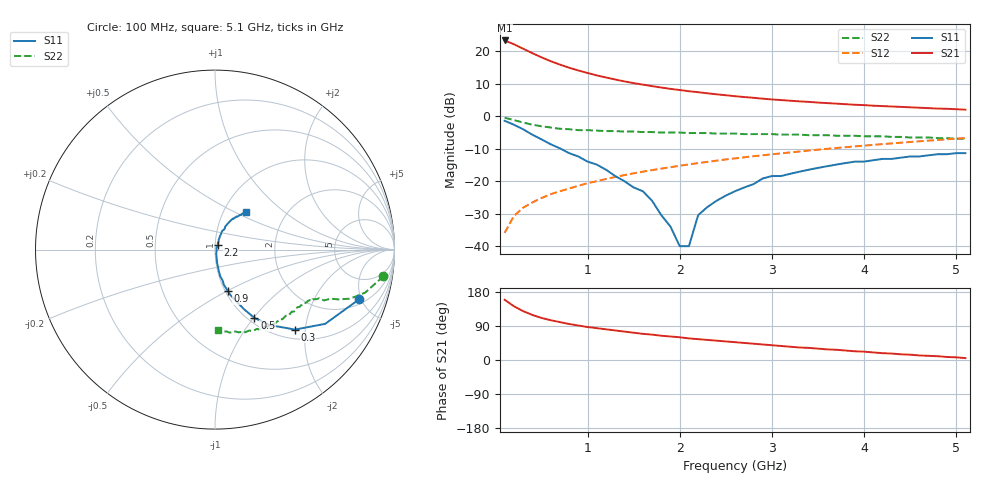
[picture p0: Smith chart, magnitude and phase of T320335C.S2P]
!AT-32033
!S PARAMETERS at Vce=5 V  Ic=5mA.  LAST UPDATED 01-05-95
# ghz s ma r 50
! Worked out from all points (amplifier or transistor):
!   51 points, 100 MHz to 5.1 GHz, reference 50 ohm
!   highest |S21| = 23.3 dB at 100 MHz (marker M1)
!   |S21| within 3 dB of that: start of sweep to 334.2 MHz
!   unconditionally stable (mu >= 1): 1.382 GHz to 2.514 GHz; 2.682 GHz to 2.705 GHz
!   at 900 MHz: K = 0.94, MSG = 17.7 dB, |S12| = -21.4 dB
!   at 2.6 GHz: K = 1.00, MSG = 9.6 dB, |S12| = -13.0 dB
!   at 5.1 GHz: K = 0.90, MSG = 4.4 dB, |S12| = -6.7 dB
!   S11 on the Smith chart (normalised r, x): 100 MHz: 2.41, -4.81; 300 MHz: 1.19, -1.76; 500 MHz: 1.07, -1.01; 900 MHz: 1.03, -0.50; 2.2 GHz: 1.03, +0.05; 5.1 GHz: 1.28, +0.57
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0.1  0.85 -19.0  14.63 159.0  0.016 79.0  0.95 -9.0
0.2  0.74 -34.0  12.81 142.0  0.029 73.0  0.87 -16.0
0.3  0.63 -45.0  10.93 129.0  0.039 69.0  0.8 -20.0
0.4  0.52 -54.0  9.34 119.0  0.047 68.0  0.74 -22.0
0.5  0.44 -60.0  8.05 111.0  0.055 67.0  0.7 -23.0
0.6  0.37 -64.0  7.02 105.0  0.063 66.0  0.67 -25.0
0.7  0.32 -67.0  6.22 100.0  0.07 66.0  0.64 -25.0
0.8  0.27 -71.0  5.57 95.0  0.077 66.0  0.63 -26.0
0.9  0.24 -73.0  5.05 91.0  0.085 66.0  0.61 -27.0
1  0.2 -76.0  4.62 87.0  0.093 66.0  0.61 -28.0
1.2  0.15 -79.0  3.94 81.0  0.108 66.0  0.59 -29.0
1.4  0.1 -80.0  3.43 75.0  0.124 66.0  0.58 -31.0
1.6  0.07 -81.0  3.06 69.0  0.14 65.0  0.57 -33.0
1.8  0.03 -76.0  2.76 64.0  0.156 64.0  0.56 -35.0
2  0.01 -17.0  2.53 60.0  0.173 63.0  0.56 -38.0
2.1  0.01 41.0  2.42 57.0  0.181 62.0  0.55 -39.0
2.2  0.03 57.0  2.34 55.0  0.19 62.0  0.55 -40.0
2.6  0.07 69.0  2.03 47.0  0.224 59.0  0.54 -46.0
2.9  0.11 69.0  1.86 41.0  0.25 56.0  0.53 -50.0
3.5  0.16 64.0  1.62 30.0  0.305 51.0  0.51 -59.0
4.3  0.22 56.0  1.41 17.0  0.381 43.0  0.48 -73.0
5.1  0.27 50.0  1.26 5.0  0.46 35.0  0.45 -88.0
